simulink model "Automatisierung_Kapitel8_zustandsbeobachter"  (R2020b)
settings: Solver=ode45  StartTime=0.0  StopTime=100  MaxStep=0.2  RelTol=1e-3  EnableMultiTasking=on
InitFcn:
  | Automatisierung_Kapitel8
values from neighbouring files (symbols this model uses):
  Ac = [0,1,0,0;-1,-1,1,1;0,0,0,1;0.1,0.1,-0.2,-0.2]    [Automatisierung_Kapitel8.m]
  AdL = Ad+kbeo'*cc    [Automatisierung_Kapitel8.m]
  AdT = Ad    [Automatisierung_Kapitel8.m]
  Bc = [bc,bvc]    [Automatisierung_Kapitel8.m]
  BdL = [bd,-kbeo']    [Automatisierung_Kapitel8.m]
  bdT = bd    [Automatisierung_Kapitel8.m]
  Cc = eye(4)    [Automatisierung_Kapitel8.m]
  CdL = eye(4)    [Automatisierung_Kapitel8.m]
  CdT = eye(4)    [Automatisierung_Kapitel8.m]
  Dc = [0,0;0,0;0,0;0,0]    [Automatisierung_Kapitel8.m]
  DdL = [0,0;0,0;0,0;0,0]    [Automatisierung_Kapitel8.m]
  ddT = [0,0,0,0]'    [Automatisierung_Kapitel8.m]
  Ta = 2    [Automatisierung_Kapitel8.m]
  x0 = [10,0,0,0]    [Automatisierung_Kapitel8.m]

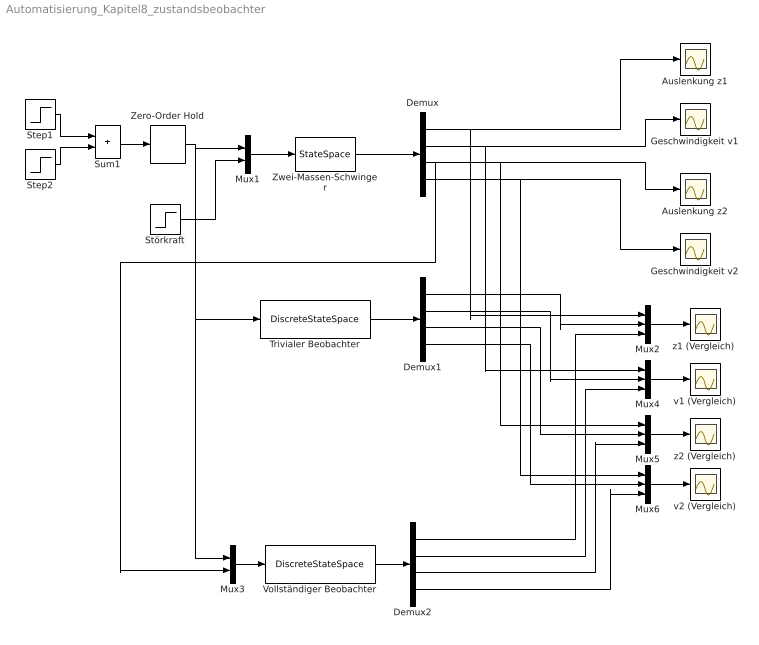
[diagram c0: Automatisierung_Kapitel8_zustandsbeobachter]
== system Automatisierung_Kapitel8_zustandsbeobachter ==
  Auslenkung z1 : Scope
  Auslenkung z2 : Scope
  Demux : Demux
  Demux1 : Demux
  Demux2 : Demux
  Geschwindigkeit v1 : Scope
  Geschwindigkeit v2 : Scope
  Mux1 : Mux  Inputs=2
  Mux{2,4..6} (4 alike) : Mux  Inputs=3
  Mux3 : Mux  Inputs=2
  Step1 : Step  Time=0  SampleTime=0
  Step2 : Step  Time=50  After=-2  SampleTime=0
  Störkraft : Step  Time=60  After=0  SampleTime=0
  Sum1 : Sum
  Trivialer Beobachter : DiscreteStateSpace  A=AdT  B=bdT  C=CdT  D=ddT  InitialCondition=[0,0,0,0]  SampleTime=Ta
  Vollständiger Beobachter : DiscreteStateSpace  A=AdL  B=BdL  C=CdL  D=DdL  InitialCondition=[0,0,0,0]  SampleTime=Ta
  Zero-Order Hold : ZeroOrderHold  SampleTime=Ta
  Zwei-Massen-Schwinger : StateSpace  A=Ac  B=Bc  C=Cc  D=Dc  InitialCondition=x0
  v1 (Vergleich) : Scope
  v2 (Vergleich) : Scope
  "z1 (Vergleich) " : Scope
  z2 (Vergleich) : Scope
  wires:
  Zwei-Massen-Schwinger/1 -> Demux/1
  Mux1/1 -> Zwei-Massen-Schwinger/1
  Zero-Order Hold/1 -> Mux1/1, Trivialer Beobachter/1, Mux3/1
  Störkraft/1 -> Mux1/2
  Demux/1 -> Auslenkung z1/1, Mux2/1
  Demux/3 -> Auslenkung z2/1, Mux5/1, Mux3/2
  Demux/2 -> Geschwindigkeit v1/1, Mux4/1
  Demux/4 -> Geschwindigkeit v2/1, Mux6/1
  Trivialer Beobachter/1 -> Demux1/1
  Demux1/1 -> Mux2/2
  Demux1/2 -> Mux4/2
  Demux1/3 -> Mux5/2
  Demux1/4 -> Mux6/2
  Mux2/1 -> "z1 (Vergleich) "/1
  Mux4/1 -> v1 (Vergleich)/1
  Mux5/1 -> z2 (Vergleich)/1
  Mux6/1 -> v2 (Vergleich)/1
  Sum1/1 -> Zero-Order Hold/1
  Step1/1 -> Sum1/1
  Step2/1 -> Sum1/2
  Mux3/1 -> Vollständiger Beobachter/1
  Vollständiger Beobachter/1 -> Demux2/1
  Demux2/1 -> Mux2/3
  Demux2/2 -> Mux4/3
  Demux2/3 -> Mux5/3
  Demux2/4 -> Mux6/3
